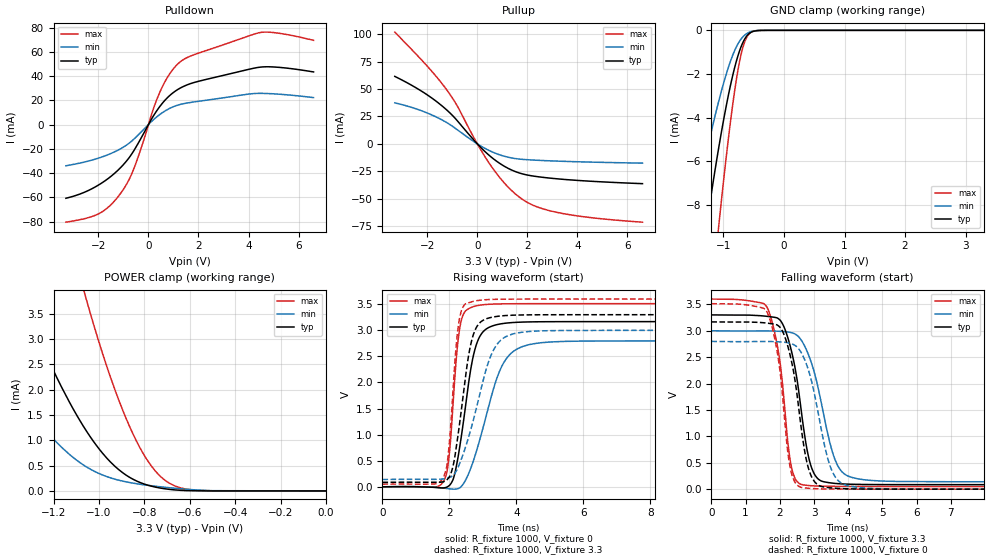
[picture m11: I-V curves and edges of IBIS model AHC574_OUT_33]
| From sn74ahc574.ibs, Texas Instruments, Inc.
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[Model]   AHC574_OUT_33
Model_type  3-state
Enable   Active-Low
Vref =   0
Rref =   1000
Cref =   50p
Vmeas =   1.65
| variable   typ   min   max
C_comp   2.06pF   1.80pF   2.21pF
| C_pullup   3.16pF   1.91pF   3.90pF
| C_pulldown   2.65pF   1.96pF   3.44pF
| C_tri-state   2.06pF   1.80pF   2.21pF
[Temperature Range]   40   100   -40
| Ambient temperature   25   85   -40
[Voltage range]   3.3   3   3.6
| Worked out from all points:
|   slope of the pulldown table from 0 to 0.495 V, typ, clamps not added: 30.9 ohm
|   slope of the pullup table from 0 to 0.495 V, typ, clamps not added: 45.5 ohm
|   GND clamp passes 1 mA (typ) near -0.74 V on its own axis
|   POWER clamp passes 1 mA (typ) near -1.03 V on its own axis
|   rising waveform, R_fixture 1000, V_fixture 0: 20-80 % time 448ps typ, 766ps min, 251ps max; typ from 0 V to 3.17 V
|   falling waveform, R_fixture 1000, V_fixture 3.3: 20-80 % time 478ps typ, 629ps min, 383ps max; typ from 3.3 V to 0.085 V
|   rising waveform, R_fixture 1000, V_fixture 3.3: 20-80 % time 416ps typ, 732ps min, 244ps max; typ from 0.085 V to 3.3 V
|   falling waveform, R_fixture 1000, V_fixture 0: 20-80 % time 448ps typ, 566ps min, 369ps max; typ from 3.17 V to 0 V
[GND Clamp]
| AHC574_OUT_33
|   Voltage   I(typ)   I(min)   I(max)
-3.3V     -60.79mA   -39.63mA   -82.28mA
-1.54V    -14.27mA   -9.073mA   -22.53mA
-1.52V    -13.84mA   -8.791mA   -21.91mA
-1.28V    -8.968mA   -5.605mA   -14.64mA
-1.1V     -5.743mA   -3.489mA   -9.559mA
-1.07V    -5.247mA   -3.165mA   -8.756mA
-905mV    -2.797mA   -1.587mA   -4.663mA
-780mV    -1.352mA   -722.8uA   -2.15mA
-690mV    -628.8uA   -334.5uA   -897.9uA
-590mV    -183.6uA   -111.4uA   -211.6uA
-375mV    -3.862uA   -2.963uA   -1.96uA
3.3V      10.71nA    15.74nA    51.49nA
[POWER Clamp]
| AHC574_OUT_33
|   Voltage   I(typ)   I(min)   I(max)
-3.3V     42.69mA    26.33mA    73.28mA
-1.61V    7.313mA    3.828mA    15.69mA
-1.36V    4.057mA    1.938mA    9.638mA
-1.205V   2.423mA    1.049mA    6.419mA
-1.07V    1.289mA    517.7uA    4.017mA
-1.055V   1.183mA    474.9uA    3.777mA
-950mV    575.2uA    259.7uA    2.258mA
-865mV    268.8uA    166.1uA    1.273mA
-790mV    120.3uA    114uA      627.9uA
-710mV    42.52uA    72.3uA     213.4uA
-570mV    2.187uA    18.48uA    12.53uA
-48.03fV  10.71nA    1.611nA    79.92nA
[Pulldown]
| AHC574_OUT_33
|   Voltage   I(typ)   I(min)   I(max)
-3.3V     -60.82mA   -34mA      -80.56mA
-1.955V   -49.36mA   -27.41mA   -73.22mA
-1.53V    -43.23mA   -24.12mA   -66.71mA
-1.095V   -35.12mA   -19.74mA   -56.23mA
-810mV    -28.34mA   -15.96mA   -46.78mA
-580mV    -21.4mA    -11.96mA   -36.16mA
195mV     7.045mA    3.905mA    12.83mA
500mV     16.14mA    8.986mA    28.77mA
890mV     24.69mA    13.77mA    43.08mA
1.32V     30.65mA    16.86mA    52.54mA
4.485V    47.4mA     25.73mA    76.01mA
6.6V      43.42mA    22.24mA    69.48mA
[Pullup]
| AHC574_OUT_33
|   Voltage   I(typ)   I(min)   I(max)
-3.3V     61.59mA    37.44mA    102mA
-2.18V    47.37mA    29.8mA     75.34mA
-1.31V    32.68mA    20.57mA    51.94mA
-830mV    21.86mA    13.38mA    35.7mA
-40mV     989.5uA    591.7uA    1.624mA
495mV     -10.88mA   -6.291mA   -18.35mA
1.08V     -20.42mA   -11.28mA   -35.71mA
1.66V     -26.4mA    -13.78mA   -48.23mA
2.305V    -29.58mA   -14.83mA   -56.72mA
3.225V    -31.92mA   -15.73mA   -62.67mA
4.605V    -34.16mA   -16.64mA   -67.43mA
6.6V      -36.27mA   -17.55mA   -71.43mA
[Ramp]
| AHC574_OUT_33
| variable   typ   min   max
dV/dt_r   1.91/4.57E-10   1.71/7.82E-10   2.11/2.55E-10
dV/dt_f   1.93/4.84E-10   1.72/6.33E-10   2.13/3.90E-10
R_load = 1000
[Rising Waveform]
| AHC574_OUT_33
R_fixture =   1000
C_fixture =   0
L_fixture =   0
V_fixture =   0
V_fixture_min = 0
V_fixture_max = 0
|   Time   V(typ)   V(min)   V(max)
0s        735.4pV    1.266nV    415.7pV
1.825ns   -21.83mV   -25.99mV   101.2mV
1.995ns   23.02mV    -38.22mV   606.8mV
2.215ns   415.1mV    -43.37mV   2.514V
2.345ns   911.3mV    -799.6uV   3.156V
2.695ns   2.447V     454.6mV    3.45V
3.005ns   2.972V     1.127V     3.491V
3.735ns   3.141V     2.484V     3.509V
5.06ns    3.166V     2.778V     3.512V
50ns      3.167V     2.798V     3.512V
[Falling Waveform]
| AHC574_OUT_33
R_fixture =   1000
C_fixture =   0
L_fixture =   0
V_fixture =   3.3
V_fixture_min = 3
V_fixture_max = 3.6
|   Time   V(typ)   V(min)   V(max)
0s        3.3V       3V         3.6V
1.635ns   3.272V     2.997V     3.437V
1.995ns   3.21V      2.99V      2.457V
2.23ns    2.88V      2.977V     921.8mV
2.34ns    2.619V     2.964V     421.2mV
2.725ns   1.028V     2.712V     77.18mV
3.035ns   260.1mV    2.149V     60.92mV
3.675ns   105.6mV    469.2mV    52.93mV
4.625ns   87.99mV    167.2mV    50.95mV
50ns      85.5mV     140.1mV    50.59mV
[Rising Waveform]
| AHC574_OUT_33
R_fixture =   1000
C_fixture =   0
L_fixture =   0
V_fixture =   3.3
V_fixture_min = 3
V_fixture_max = 3.6
|   Time   V(typ)   V(min)   V(max)
0s        85.5mV     140.1mV    50.59mV
1.82ns    95.99mV    151.3mV    176.1mV
1.97ns    163.3mV    170.9mV    639.5mV
2.195ns   707.8mV    289.2mV    2.637V
2.31ns    1.234V     452.8mV    3.246V
2.62ns    2.672V     1.052V     3.537V
2.93ns    3.158V     1.83V      3.579V
3.5ns     3.274V     2.788V     3.596V
4.675ns   3.299V     2.988V     3.6V
50ns      3.3V       3V         3.6V
[Falling Waveform]
| AHC574_OUT_33
R_fixture =   1000
C_fixture =   0
L_fixture =   0
V_fixture =   0
V_fixture_min = 0
V_fixture_max = 0
|   Time   V(typ)   V(min)   V(max)
0s        3.167V     2.798V     3.512V
1.63ns    3.144V     2.797V     3.351V
1.96ns    3.094V     2.791V     2.458V
2.215ns   2.753V     2.774V     806.7mV
2.385ns   2.287V     2.744V     214.3mV
2.715ns   769.2mV    2.47V      24.13mV
3ns       156.3mV    1.843V     10.15mV
3.53ns    22.44mV    341.5mV    2.906mV
4.425ns   2.914mV    25.1mV     504.2uV
50ns      852.6pV    8.864nV    -2.235nV
